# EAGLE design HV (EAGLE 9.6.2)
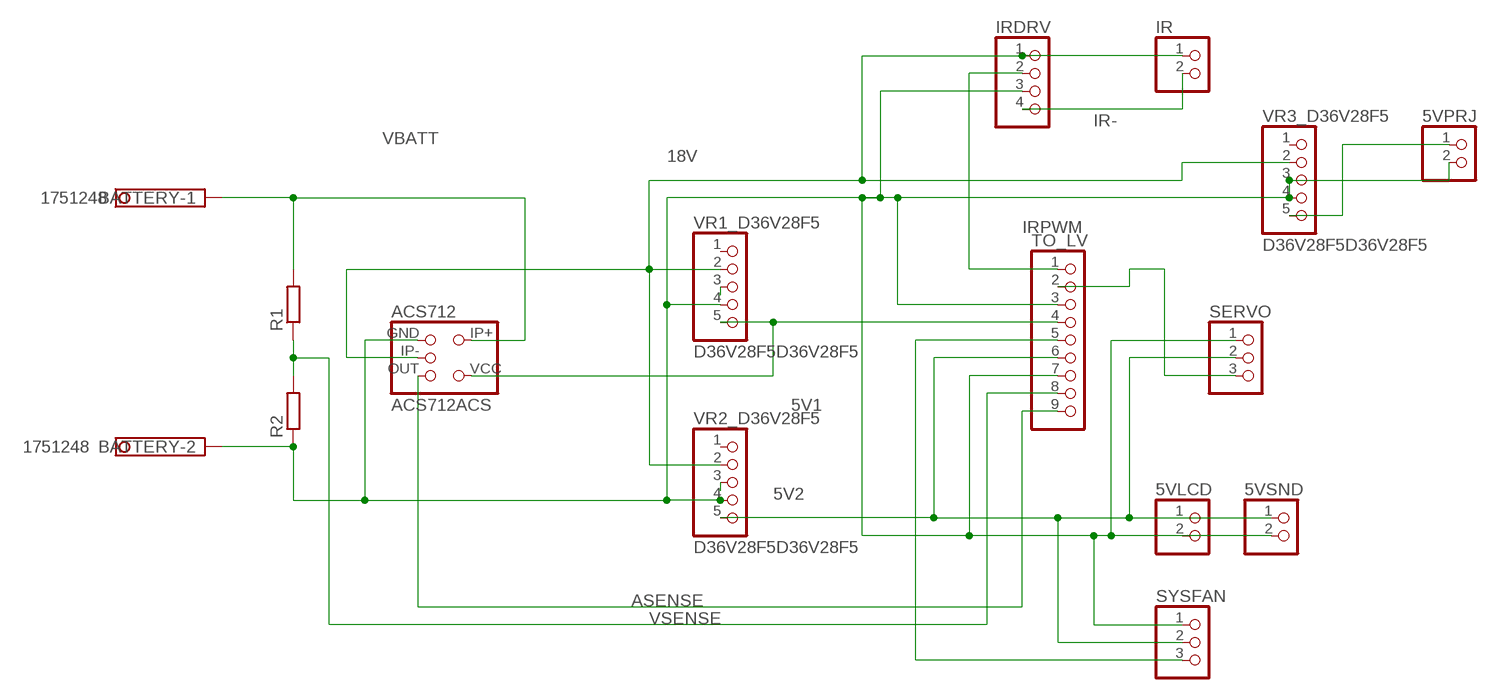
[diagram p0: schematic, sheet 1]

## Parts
5VLCD  PINHD-1X2  [1X02]
5VPRJ  PINHD-1X2  [1X02]
5VSND  PINHD-1X2  [1X02]
ACS712  ACS712ACS  [DIP2400W53P254L1969H508Q6B]
BATTERY  1751248  [1751248]
IR  PINHD-1X2  [1X02]
IRDRV  PINHD-1X4  [1X04]
R1  R-EU_0204/7  [0204/7]
R2  R-EU_0204/7  [0204/7]
SERVO  PINHD-1X3  [1X03]
SYSFAN  PINHD-1X3  [1X03]
TO_LV  THROUGHCON  [THROUGH]
VR1_D36V28F5  D36V28F5D36V28F5  [DIP762W53P254L1969H508Q16B]
VR2_D36V28F5  D36V28F5D36V28F5  [DIP762W53P254L1969H508Q16B]
VR3_D36V28F5  D36V28F5D36V28F5  [DIP762W53P254L1969H508Q16B]

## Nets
5V1: ACS712.VCC TO_LV.4 VR1_D36V28F5.5
5V2: 5VLCD.1 5VSND.1 SERVO.2 SYSFAN.2 TO_LV.6 VR2_D36V28F5.5
5VPRJ: 5VPRJ.1 VR3_D36V28F5.5
18V [18VPWR]: ACS712.IP- IR.1 IRDRV.1 VR1_D36V28F5.2 VR2_D36V28F5.2 VR3_D36V28F5.2
ASENSE: ACS712.OUT TO_LV.9
FANPWM: SYSFAN.3 TO_LV.5
GND [18VPWR]: 5VLCD.2 5VPRJ.2 5VSND.2 ACS712.GND BATTERY.2 IRDRV.3 R2.1 SERVO.1 SYSFAN.1 TO_LV.3 TO_LV.7 VR1_D36V28F5.4 VR2_D36V28F5.4 VR3_D36V28F5.3 VR3_D36V28F5.4
IR-: IR.2 IRDRV.4
IRPWM: IRDRV.2 TO_LV.1
N$1 [18VPWR]: VR1_D36V28F5.3
N$2 [18VPWR]: VR2_D36V28F5.3
SERVOPWM: SERVO.3 TO_LV.2
VBATT [18VPWR]: ACS712.IP+ BATTERY.1 R1.2
VSENSE: R1.1 R2.2 TO_LV.8
Unconnected: VR1_D36V28F5.1 VR2_D36V28F5.1 VR3_D36V28F5.1

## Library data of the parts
5VLCD 5VPRJ 5VSND IR = pinhead:PINHD-1X2: PIN HEADER
ACS712 = raspberrypi_bastelstube_v13:ACS712
BATTERY = con-phoenix-350:1751248: MKDS 1/ 2-3,5 Printklemme; OC_FARNELL: unknown; OC_NEWARK: unknown
IRDRV = pinhead:PINHD-1X4: PIN HEADER
R1 R2 = rcl:R-EU_: RESISTOR, European symbol; SPICEPREFIX: R
SERVO SYSFAN = pinhead:PINHD-1X3: PIN HEADER
TO_LV = raspberrypi_bastelstube_v13:THROUGHCON
VR1_D36V28F5 VR2_D36V28F5 VR3_D36V28F5 = raspberrypi_bastelstube_v13:D36V28F5

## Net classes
0 default: width 1.5 mm, clearance 0.508 mm
1 18VPWR: width 2 mm, clearance 0.508 mm

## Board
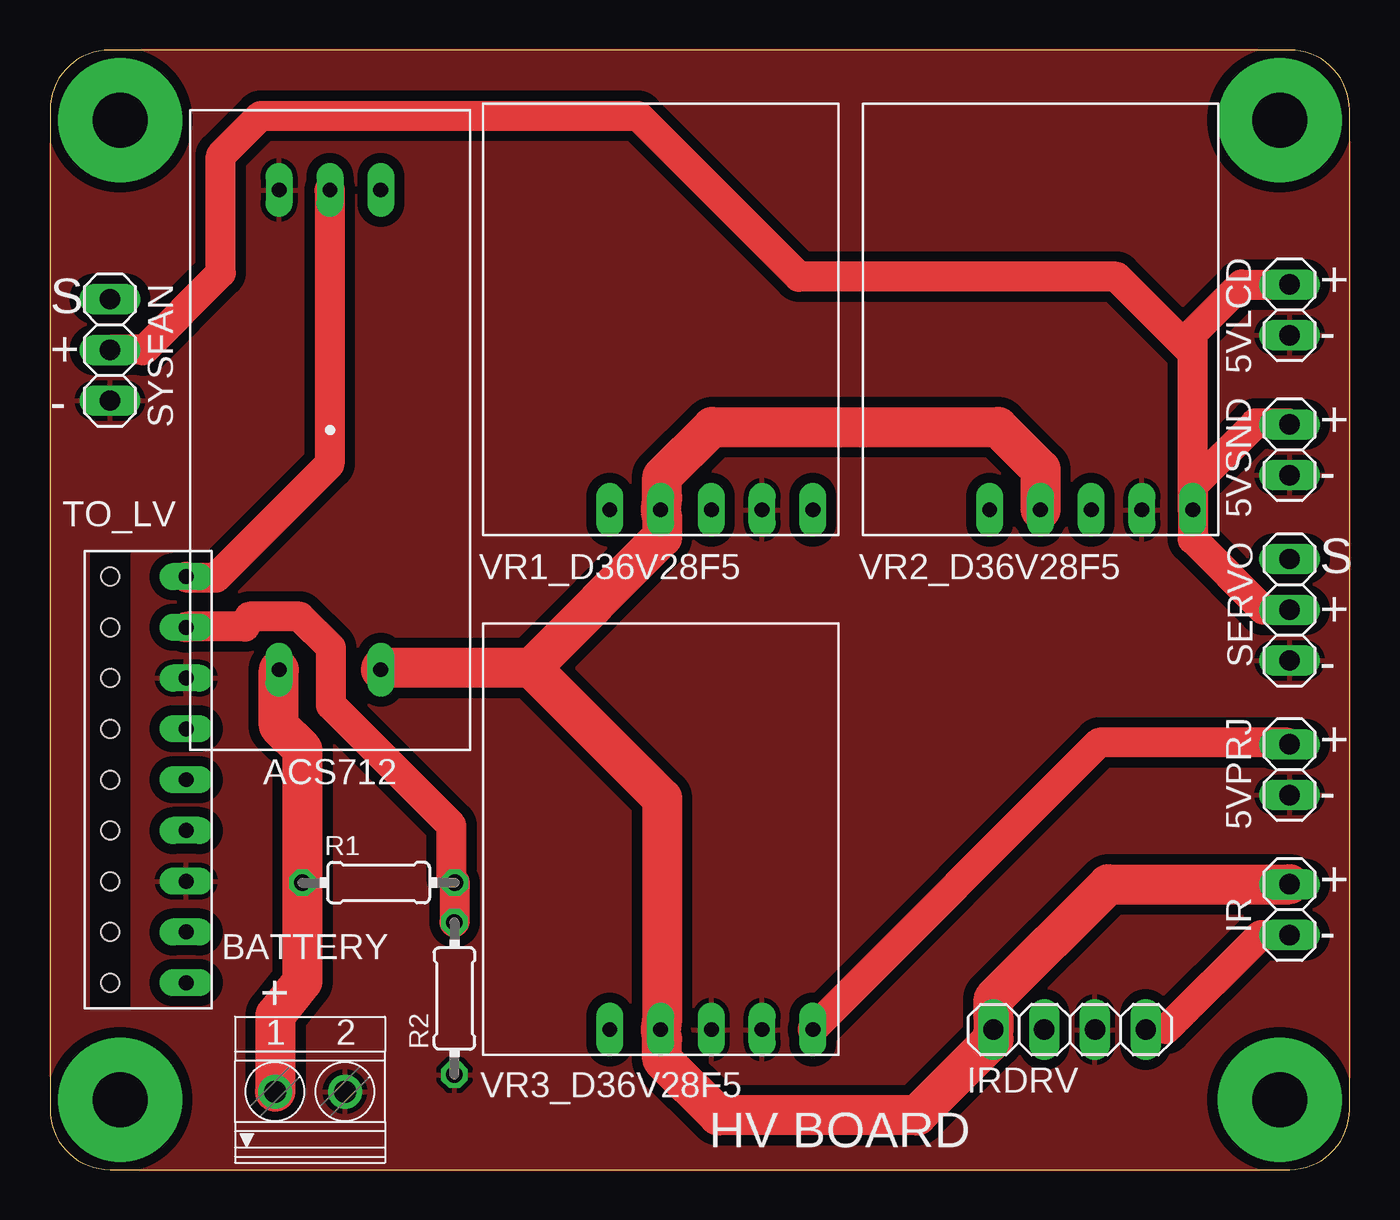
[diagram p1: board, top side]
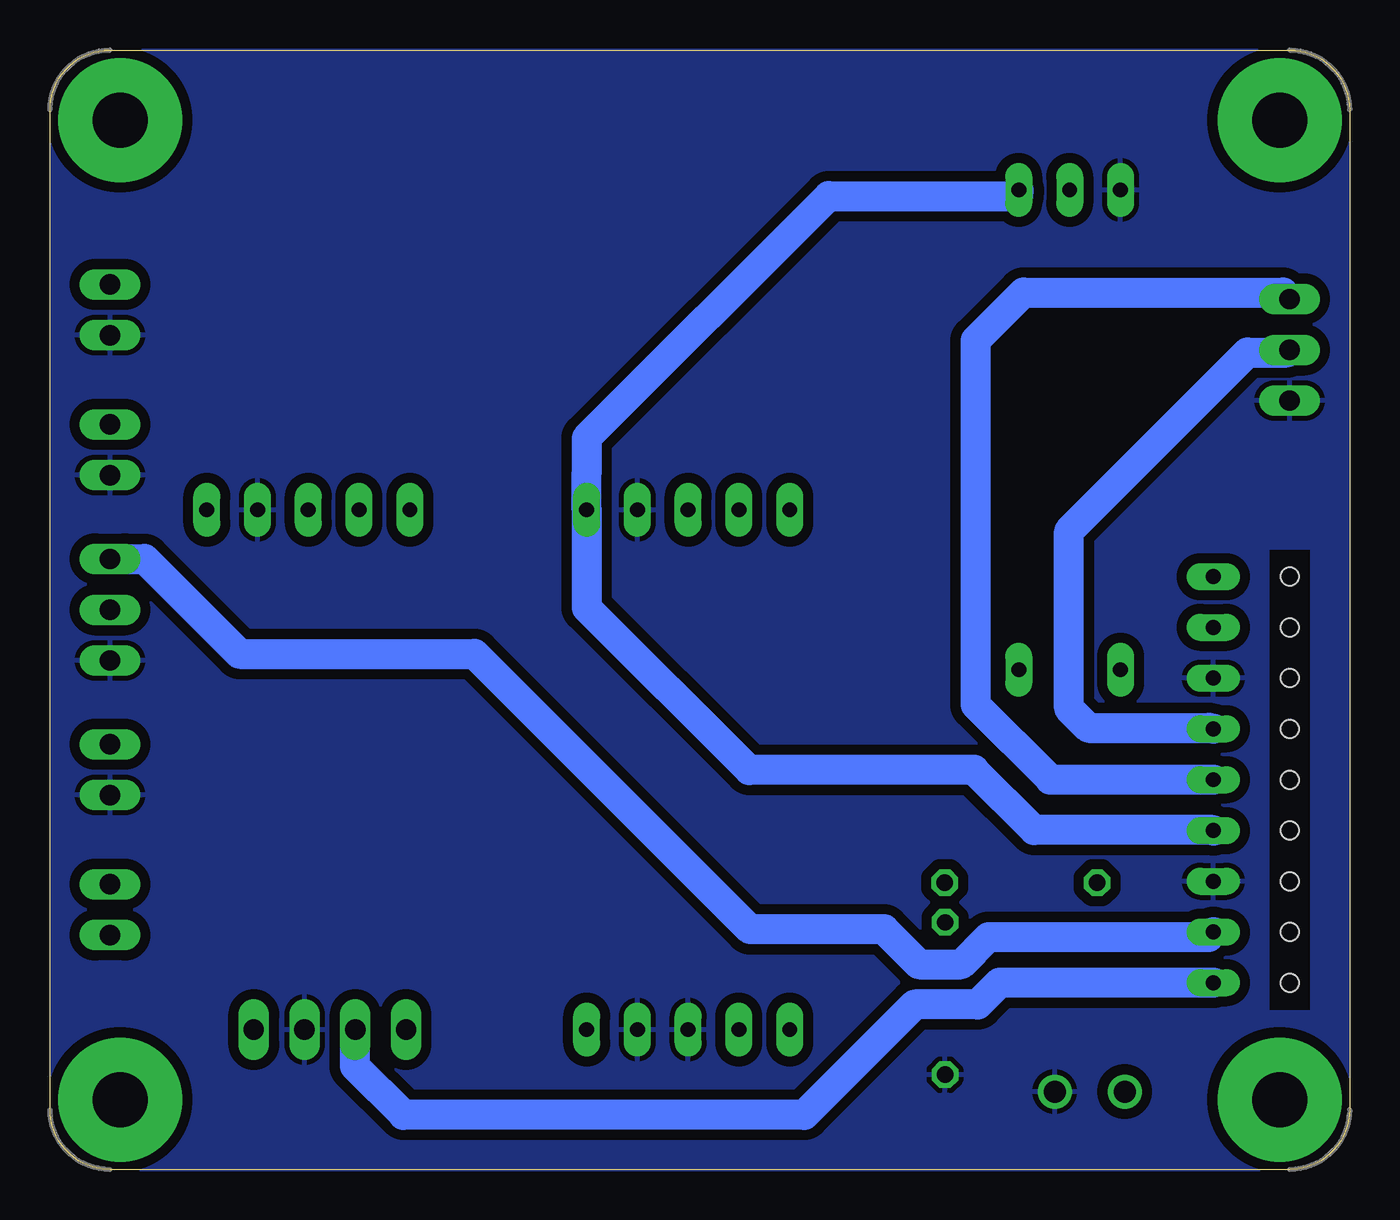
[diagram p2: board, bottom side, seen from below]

Size 65 x 56 mm. Coordinates in mm from the lower left corner, seen from the top.
Outline: 0,53 0,3 arc90 3,0 62,0 arc90 65,3 65,53 arc90 62,56 3,56 arc90 0,53
Copper layers (1*16): Top 0.035mm / dielectric 1.5mm / Bottom 0.035mm
Design rules "default *": minimum track width 6mil, minimum drill 0.35mm, track to track 6mil, track to pad 6mil, pad to pad 6mil, via to via 6mil, smd to smd 6mil, copper to edge 0mil, drill to drill 6mil, minimum pad ring 10mil, minimum via ring 8mil, stop-mask expansion 4mil, vias tented up to drill 0mil, thermal gap 10mil
tRestrict: area 2,8 to 4,31
bRestrict: area 2,8 to 4,31

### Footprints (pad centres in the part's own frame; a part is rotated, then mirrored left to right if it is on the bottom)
1X02 = drill 1.016 long: 1 -1.27,0; 2 1.27,0
DIP2400W53P254L1969H508Q6B = drill 0.743 pad 1.343 long: GND 2.54,-12; IP+ 2.54,12; IP- -2.54,12; OUT 0,-12; VCC -2.54,-12
1751248 = drill 1.1 pad 1.7: 1 -1.75,-0.1; 2 1.75,-0.1
1X04 = drill 1.016 long: 1 -3.81,0; 2 -1.27,0; 3 1.27,0; 4 3.81,0
0204/7 = drill 0.813 octagon: 1 -3.81,0; 2 3.81,0
1X03 = drill 1.016 long: 1 -2.54,0; 2 0,0; 3 2.54,0
THROUGH = drill 0.743 pad 1.343 long: 1 -10.16,-3.81; 2 -7.62,-3.81; 3 -5.08,-3.81; 4 -2.54,-3.81; 5 0,-3.81; 6 2.54,-3.81; 7 5.08,-3.81; 8 7.62,-3.81; 9 10.16,-3.81 | hole 0.9: 0,0; -2.54,0; -5.08,0; -7.62,0; -10.16,0; 2.54,0; 5.08,0; 7.62,0; 10.16,0
PWR = drill 2.75 pad 6.2: 41 3.5,3.5; 42 61.5,3.5; 43 61.5,52.5; 44 3.5,52.5
DIP762W53P254L1969H508Q16B = drill 0.743 pad 1.343 long: 1 0,0; 2 2.54,0; 3 5.08,0; 4 7.62,0; 5 10.16,0

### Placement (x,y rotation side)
5VLCD  62,43 270 top
5VPRJ  62,20 270 top
5VSND  62,36 270 top
ACS712  14,37 180 top
BATTERY  13,4 0 top
IR  62,13 270 top
IRDRV  51,7 0 top
R1  16.44,14.35 180 top
R2  20.23,8.56 90 top
SERVO  62,28 90 top
SYSFAN  3,41 90 top
TO_LV  3,19.5 90 top
U$2  PWR  [PWR]  0,0 0 top
VR1_D36V28F5  28,33 0 top
VR2_D36V28F5  47,33 0 top
VR3_D36V28F5  28,7 0 top

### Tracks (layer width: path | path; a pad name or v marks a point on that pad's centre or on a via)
5V1
  Bottom 1.5: ACS712.VCC 16.57,48.69 26.04,48.69 38.15,36.58 38.15,34.89 38.16,34.88 VR1_D36V28F5.5 38.16,28.11 30.02,19.98 30,20 18.78,20 15.76,16.98 6.83,16.98 TO_LV.4
5V2
  Top 1.5: SERVO.2 60.69,28 57.16,31.53 VR2_D36V28F5.5 | 5VSND.1 61.95,37.32 60.28,37.32 57.16,34.2 VR2_D36V28F5.5 | SYSFAN.2 4.61,41.01 4.66,40.97 8.54,44.86 8.54,50.71 10.54,52.71 29.4,52.71 37.45,44.65 53.35,44.65 57.16,40.84 | 57.16,40.84 57.16,41.83 59.6,44.27 5VLCD.1 | VR2_D36V28F5.5 57.16,40.84
  Bottom 1.5: TO_LV.6 7.03,22.09 13.05,22.09 14.03,23.07 14.03,31.93 5.1,40.87 3.13,40.87 SYSFAN.2
5VPRJ
  Top 1.5: VR3_D36V28F5.5 38.16,7.02 52.5,21.36 61.88,21.36 5VPRJ.1
18V
  Top 2: IR.1 52.93,14.27 47.19,8.53 47.19,7.53 IRDRV.1 47.19,6.53 43.37,2.71 33.44,2.71 30.62,5.52 30.62,6.53 VR3_D36V28F5.2 30.62,7.53 30.62,18.57 24.1,25.1 | 24.1,25.1 16.57,25.1 ACS712.IP- | 24.1,25.1 30.62,31.63 30.62,32.63 VR1_D36V28F5.2 30.62,33.63 30.62,34.64 33.13,37.14 47.41,37.14 49.55,35.01 VR2_D36V28F5.2
ASENSE
  Top 1.5: TO_LV.9 6.87,29.6 8.29,29.6 13.98,35.29 13.98,48.98 ACS712.OUT
FANPWM
  Bottom 1.5: SYSFAN.3 3.33,43.87 16.31,43.87 18.7,41.47 18.7,23.24 14.97,19.51 6.83,19.51 TO_LV.5
GND
  pour Bottom: 62,0 3,0 arc-90 0,3 0,53 arc-90 3,56 62,56 arc-90 65,53 65,3 arc-90
  pour Top: 0,53 0,3 arc90 3,0 62,0 arc90 65,3 65,53 arc90 62,56 3,56 arc90
IR-
  Top 1.5: IRDRV.4 55.22,7.03 55.83,7.03 60.43,11.62 60.58,11.73 IR.2
IRPWM
  Bottom 1.5: TO_LV.1 17.51,9.34 18.59,8.26 21.74,8.26 27.27,2.73 47.32,2.73 49.76,5.17 49.76,6.97 IRDRV.2
SERVOPWM
  Bottom 1.5: SERVO.3 60.27,30.54 55.52,25.8 43.77,25.8 29.99,12.01 23.28,12.01 21.54,10.27 19.42,10.27 18.06,11.63 7.06,11.63 TO_LV.2
VBATT
  Top 2: BATTERY.1 11.28,3.91 11.28,7.72 12.63,9.41 R1.2 12.63,21.01 11.44,22.2 11.44,24.98 ACS712.IP+
VSENSE
  Top 1.5: R2.2 20.25,12.42 R1.1 20.08,14.59 20.08,17.21 14.06,23.23 14.06,26.1 12.5,27.66 9.98,27.66 9.76,27.16 6.85,27.16 TO_LV.8

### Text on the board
tNames: + / - | S / + / - | + / - | S / + / - | + / - | + / - | + | HV BOARD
